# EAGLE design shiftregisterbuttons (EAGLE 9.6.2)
Assembly variants: CS HIGH, CS LOW
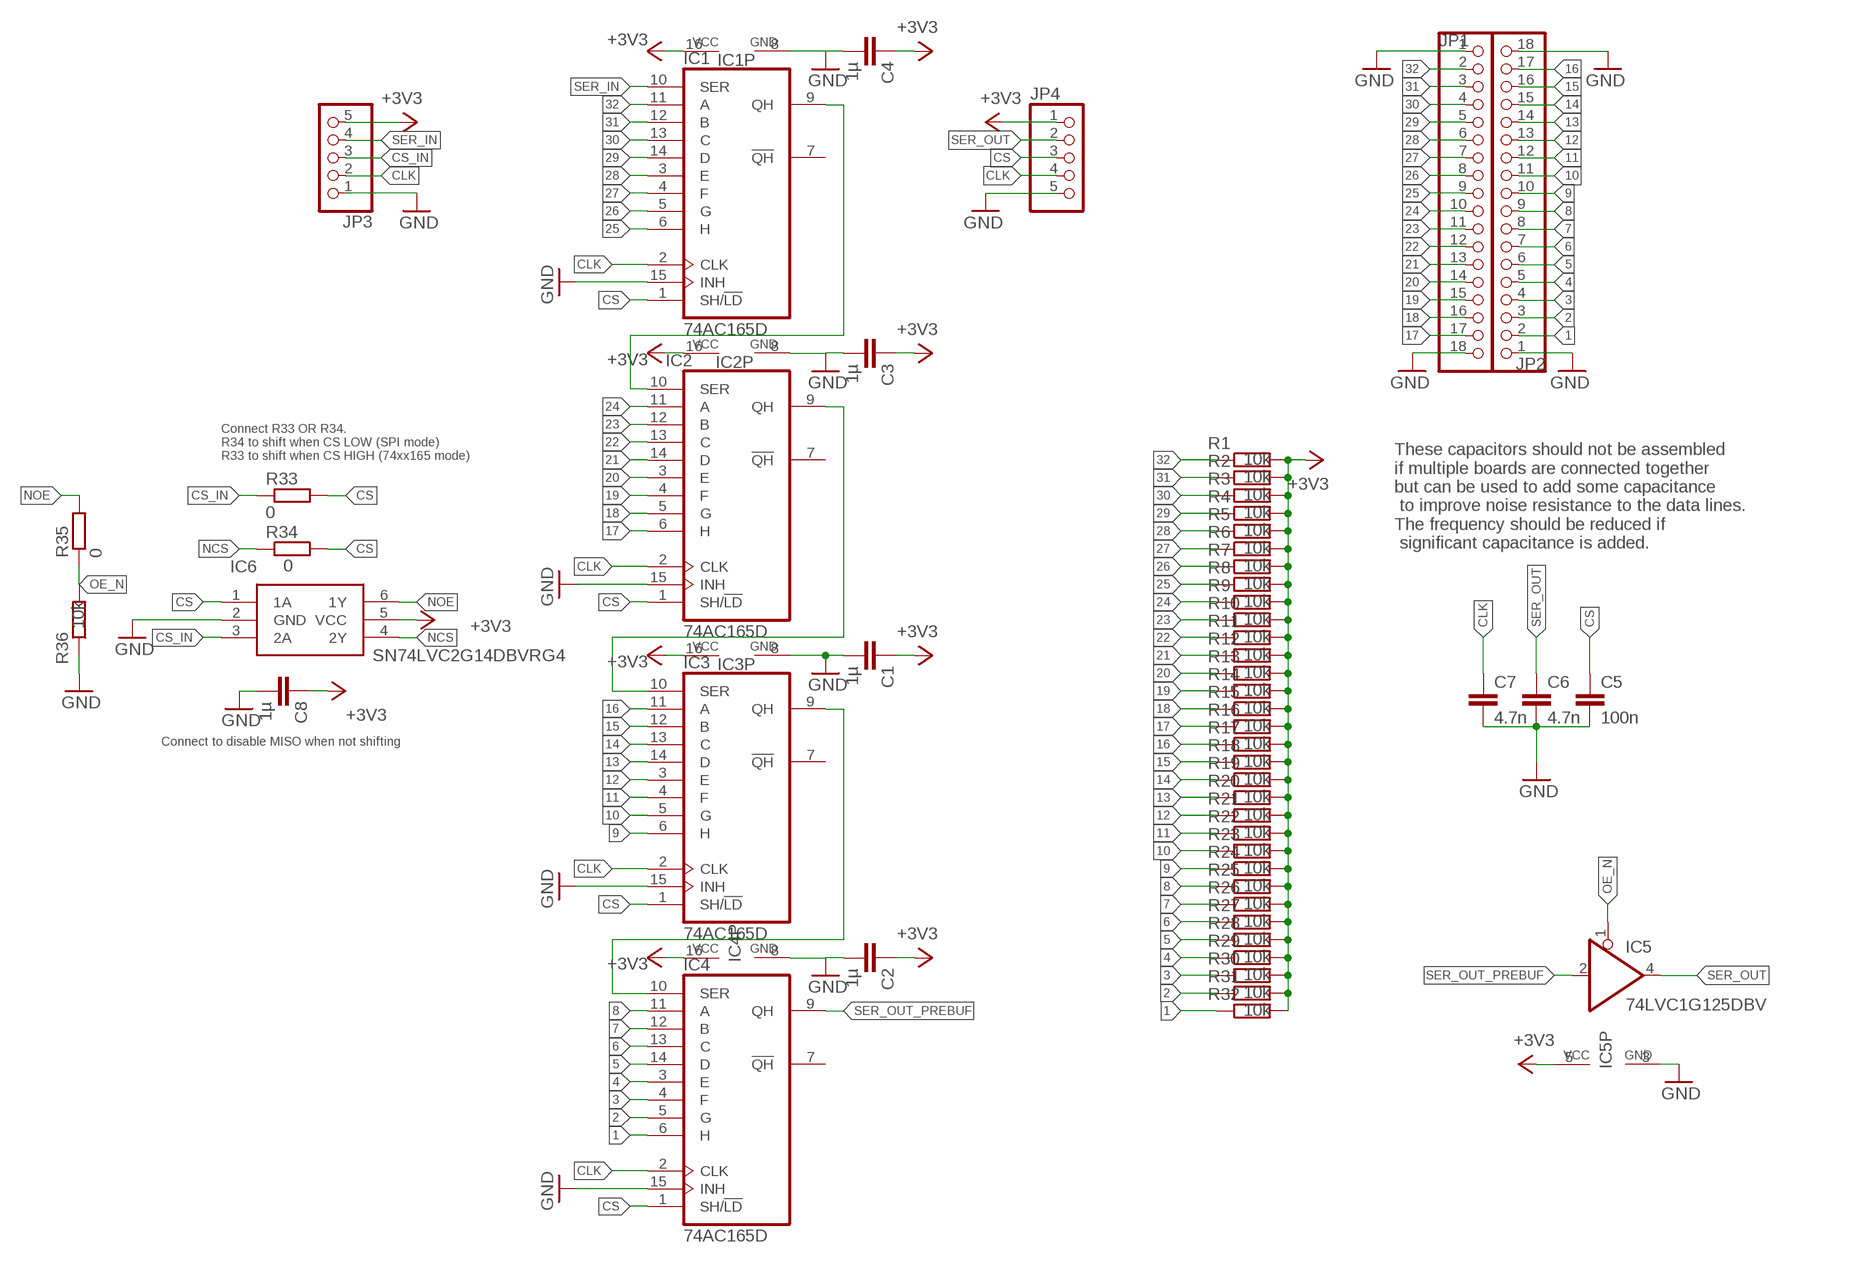
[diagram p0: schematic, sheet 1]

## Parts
C1  1µ  C-EUC0603  [C0603]
C2  1µ  C-EUC0603  [C0603]
C3  1µ  C-EUC0603  [C0603]
C4  1µ  C-EUC0603  [C0603]
C5  100n  C-EUC0603  [C0603]  (not fitted in variant CS HIGH)  (not fitted in variant CS LOW)
C6  4.7n  C-EUC0603  [C0603]  (not fitted in variant CS HIGH)  (not fitted in variant CS LOW)
C7  4.7n  C-EUC0603  [C0603]  (not fitted in variant CS HIGH)  (not fitted in variant CS LOW)
C8  1µ  C-EUC0603  [C0603]
IC1  74AC165D  [SO16]
IC2  74AC165D  [SO16]
IC3  74AC165D  [SO16]
IC4  74AC165D  [SO16]
IC5  74LVC1G125DBV  [SOT23-5]
IC6  SN74LVC2G14DBVRG4  [SOT95P280X145-6N]
JP1  PINHD-1X18  [1X18]
JP2  PINHD-1X18  [1X18]
JP3  PINHD-1X5  [1X05]
JP4  PINHD-1X5  [1X05]
R1  10k  R-EU_R0603  [R0603]
R2  10k  R-EU_R0603  [R0603]
R3  10k  R-EU_R0603  [R0603]
R4  10k  R-EU_R0603  [R0603]
R5  10k  R-EU_R0603  [R0603]
R6  10k  R-EU_R0603  [R0603]
R7  10k  R-EU_R0603  [R0603]
R8  10k  R-EU_R0603  [R0603]
R9  10k  R-EU_R0603  [R0603]
R10  10k  R-EU_R0603  [R0603]
R11  10k  R-EU_R0603  [R0603]
R12  10k  R-EU_R0603  [R0603]
R13  10k  R-EU_R0603  [R0603]
R14  10k  R-EU_R0603  [R0603]
R15  10k  R-EU_R0603  [R0603]
R16  10k  R-EU_R0603  [R0603]
R17  10k  R-EU_R0603  [R0603]
R18  10k  R-EU_R0603  [R0603]
R19  10k  R-EU_R0603  [R0603]
R20  10k  R-EU_R0603  [R0603]
R21  10k  R-EU_R0603  [R0603]
R22  10k  R-EU_R0603  [R0603]
R23  10k  R-EU_R0603  [R0603]
R24  10k  R-EU_R0603  [R0603]
R25  10k  R-EU_R0603  [R0603]
R26  10k  R-EU_R0603  [R0603]
R27  10k  R-EU_R0603  [R0603]
R28  10k  R-EU_R0603  [R0603]
R29  10k  R-EU_R0603  [R0603]
R30  10k  R-EU_R0603  [R0603]
R31  10k  R-EU_R0603  [R0603]
R32  10k  R-EU_R0603  [R0603]
R33  0  R-EU_R0603  [R0603]  (not fitted in variant CS LOW)
R34  0  R-EU_R0603  [R0603]  (not fitted in variant CS HIGH)
R35  0  R-EU_R0603  [R0603]
R36  10k  R-EU_R0603  [R0603]

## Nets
1: IC4.6(H) JP2.2 R32.1
2: IC4.5(G) JP2.3 R31.1
3: IC4.4(F) JP2.4 R30.1
4: IC4.3(E) JP2.5 R29.1
5: IC4.14(D) JP2.6 R28.1
6: IC4.13(C) JP2.7 R27.1
7: IC4.12(B) JP2.8 R26.1
8: IC4.11(A) JP2.9 R25.1
9: IC3.6(H) JP2.10 R24.1
10: IC3.5(G) JP2.11 R23.1
11: IC3.4(F) JP2.12 R22.1
12: IC3.3(E) JP2.13 R21.1
13: IC3.14(D) JP2.14 R20.1
14: IC3.13(C) JP2.15 R19.1
15: IC3.12(B) JP2.16 R18.1
16: IC3.11(A) JP2.17 R17.1
17: IC2.6(H) JP1.17 R16.1
18: IC2.5(G) JP1.16 R15.1
19: IC2.4(F) JP1.15 R14.1
20: IC2.3(E) JP1.14 R13.1
21: IC2.14(D) JP1.13 R12.1
22: IC2.13(C) JP1.12 R11.1
23: IC2.12(B) JP1.11 R10.1
24: IC2.11(A) JP1.10 R9.1
25: IC1.6(H) JP1.9 R8.1
26: IC1.5(G) JP1.8 R7.1
27: IC1.4(F) JP1.7 R6.1
28: IC1.3(E) JP1.6 R5.1
29: IC1.14(D) JP1.5 R4.1
30: IC1.13(C) JP1.4 R3.1
31: IC1.12(B) JP1.3 R2.1
32: IC1.11(A) JP1.2 R1.1
+3V3: C1.1 C2.1 C3.1 C4.1 C8.1 IC1.16(VCC) IC2.16(VCC) IC3.16(VCC) IC4.16(VCC) IC5.5(VCC) IC6.5(VCC) JP3.5 JP4.1 R1.2 R2.2 R3.2 R4.2 R5.2 R6.2 R7.2 R8.2 R9.2 R10.2 R11.2 R12.2 R13.2 R14.2 R15.2 R16.2 R17.2 R18.2 R19.2 R20.2 R21.2 R22.2 R23.2 R24.2 R25.2 R26.2 R27.2 R28.2 R29.2 R30.2 R31.2 R32.2
CLK: C7.1 IC1.2(CLK) IC2.2(CLK) IC3.2(CLK) IC4.2(CLK) JP3.2 JP4.4
CS: C5.1 IC1.1(SH/!LD) IC2.1(SH/!LD) IC3.1(SH/!LD) IC4.1(SH/!LD) IC6.1(1A) JP4.3 R33.2 R34.2
CS_IN: IC6.3(2A) JP3.3 R33.1
GND: C1.2 C2.2 C3.2 C4.2 C5.2 C6.2 C7.2 C8.2 IC1.8(GND) IC1.15(INH) IC2.8(GND) IC2.15(INH) IC3.8(GND) IC3.15(INH) IC4.8(GND) IC4.15(INH) IC5.3(GND) IC6.2(GND) JP1.1 JP1.18 JP2.1 JP2.18 JP3.1 JP4.5 R36.1
N$1: IC2.9(QH) IC3.10(SER)
N$2: IC3.9(QH) IC4.10(SER)
NCS: IC6.4(2Y) R34.1
NOE: IC6.6(1Y) R35.2
OE_N: IC5.1(OE) R35.1 R36.2
SER1: IC1.9(QH) IC2.10(SER)
SER_IN: IC1.10(SER) JP3.4
SER_OUT: C6.1 IC5.4(O) JP4.2
SER_OUT_PREBUF: IC4.9(QH) IC5.2(I)
Unconnected: IC1.7(!QH) IC2.7(!QH) IC3.7(!QH) IC4.7(!QH)

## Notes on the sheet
- Connect R33 OR R34.
  R34 to shift when CS LOW (SPI mode)
  R33 to shift when CS HIGH (74xx165 mode)
- These capacitors should not be assembled 
  if multiple boards are connected together 
  but can be used to add some capacitance
   to improve noise resistance to the data lines.
  The frequency should be reduced if
   significant capacitance is added.
- Connect to disable MISO when not shifting

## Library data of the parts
C1-C8 = resistor:C-EU: CAPACITOR, European symbol
IC1-IC4 = 74xx-eu:74*165: 8-bit parallel load SHIFT REGISTER
IC5 = 74xx-little-de:74*1G125: Single Bus Buffer Gate with 3-State Output
IC6 = SamacSys_Parts:SN74LVC2G14DBVRG4: Dual Schmitt-Trigger Inverter Source: Datasheet; ARROW_PART_NUMBER: SN74LVC2G14DBVRG4; ARROW_PRICE-STOCK: https://www.arrow.com/en/products/sn74lvc2g14dbvrg4/texas-instruments?utm_currency=USD&region=nac; DESCRIPTION: Dual Schmitt-Trigger Inverter; HEIGHT: 1.45mm; MANUFACTURER_NAME: Texas Instruments; MANUFACTURER_PART_NUMBER: SN74LVC2G14DBVRG4; MOUSER_PART_NUMBER: 595-SN74LVC2G14DBVG4; MOUSER_PRICE-STOCK: https://www.mouser.co.uk/ProductDetail/Texas-Instruments/SN74LVC2G14DBVRG4?qs=pajgIaoyDUjLahZkznp%2F9Q%3D%3D
JP1 JP2 = pinhead:PINHD-1X18: PIN HEADER
JP3 JP4 = pinhead:PINHD-1X5: PIN HEADER
R1-R36 = resistor:R-EU_: RESISTOR, European symbol

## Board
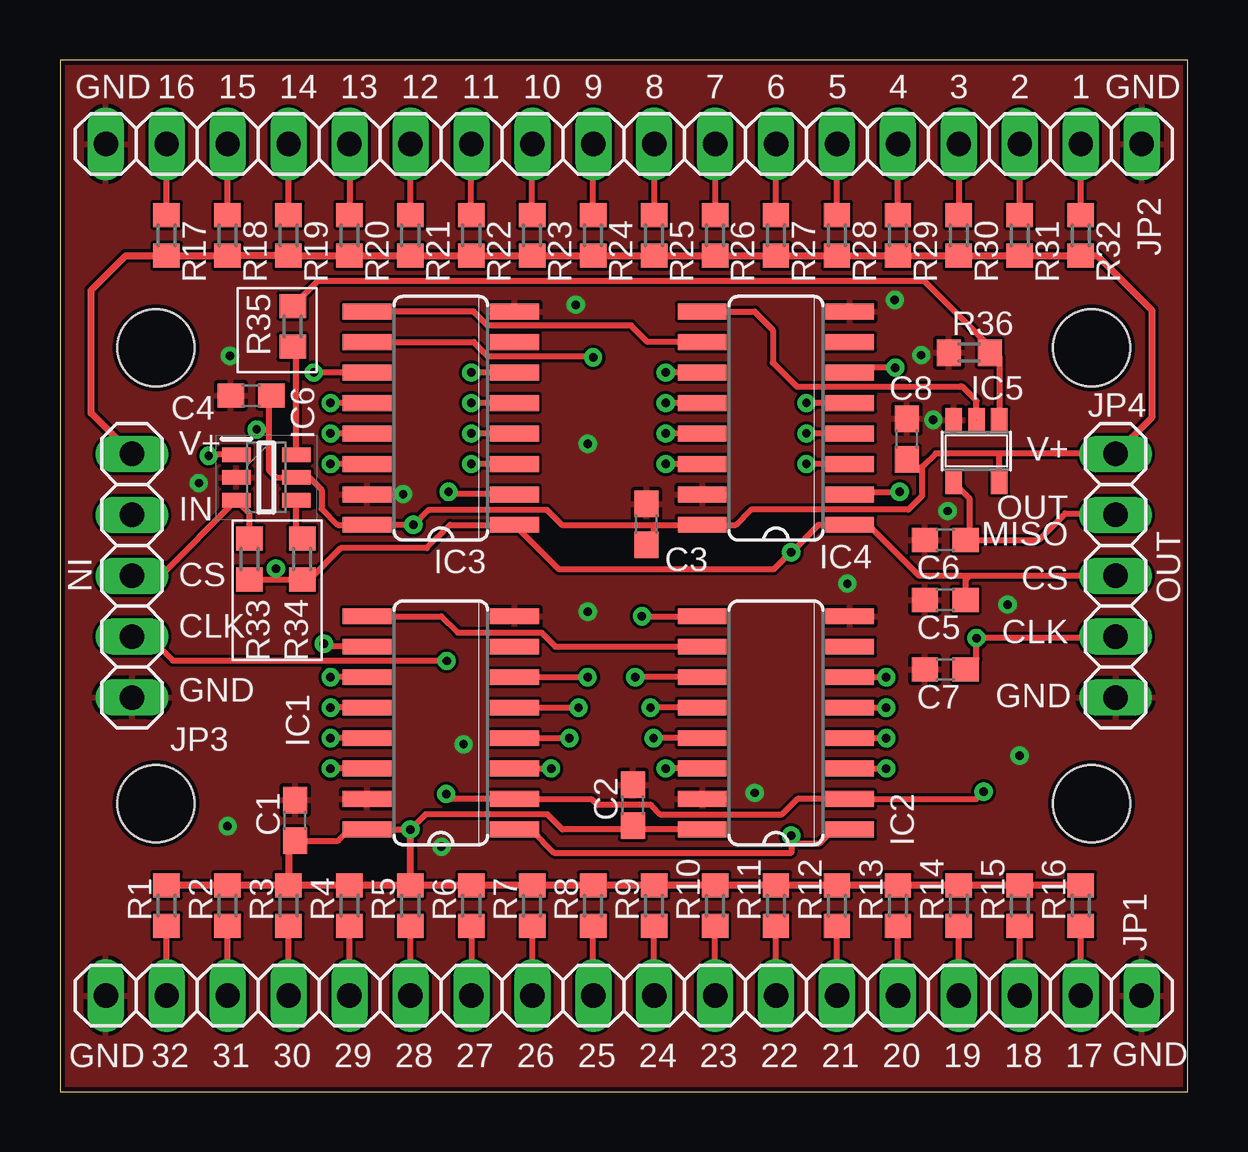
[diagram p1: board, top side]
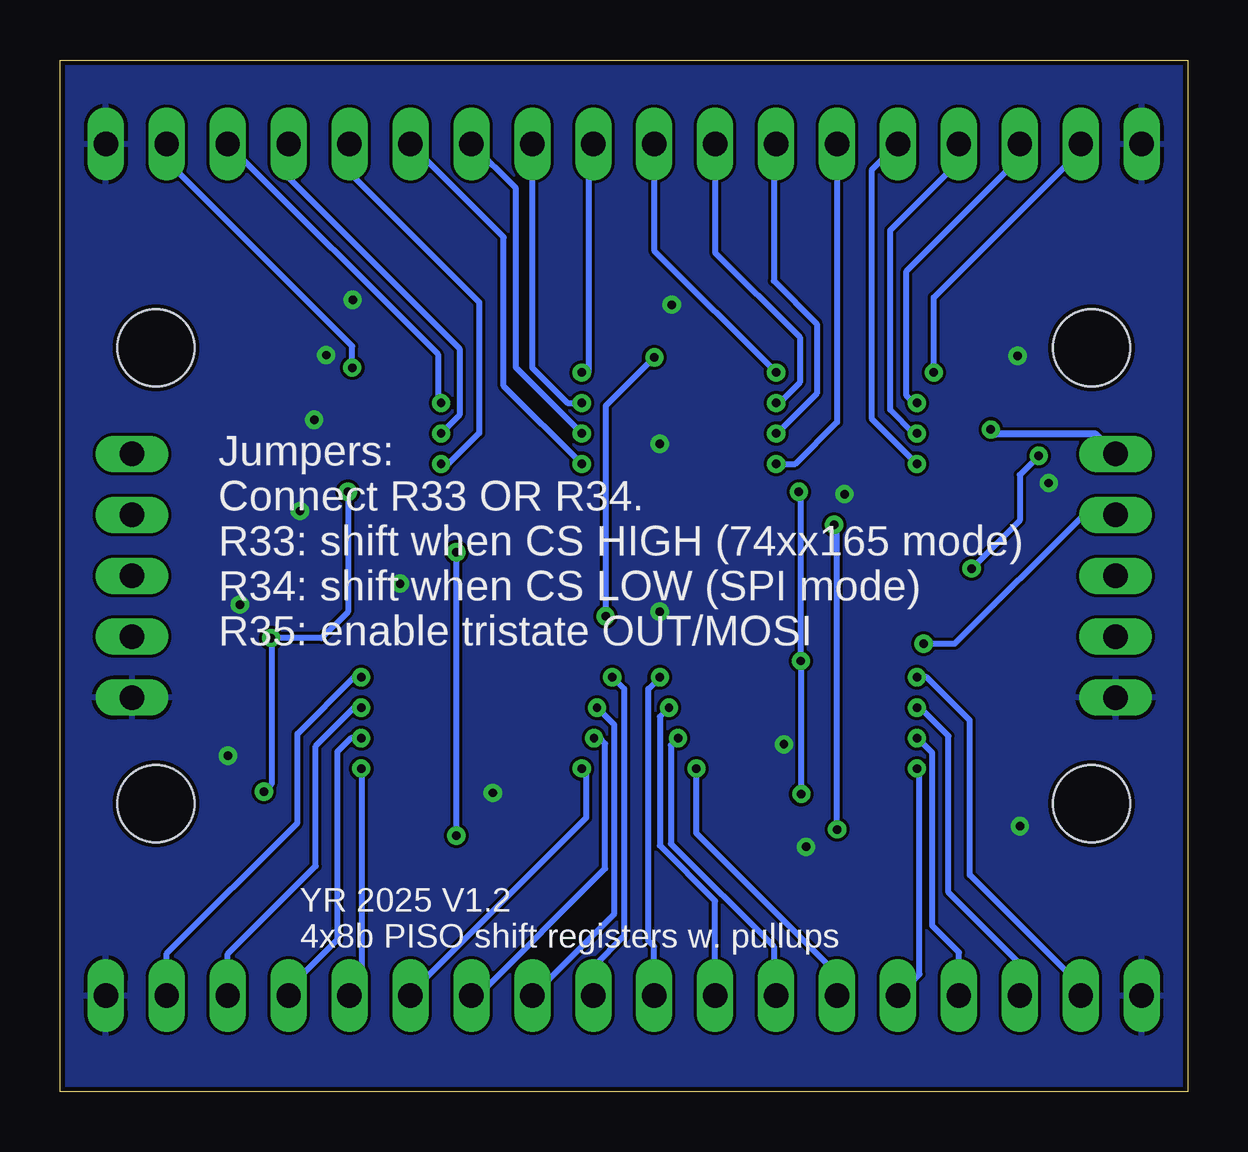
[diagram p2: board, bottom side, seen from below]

Size 47 x 43 mm. Coordinates in mm from the lower left corner, seen from the top.
Outline: 0,43 0,0 47,0 47,43 0,43
Copper layers (1*16): Top 0.035mm / dielectric 1.5mm / Bottom 0.035mm
Design rules "jlcpcb *": minimum track width 5mil, minimum drill 0.3mm, track to track 5mil, track to pad 5mil, pad to pad 5mil, via to via 5mil, smd to smd 5mil, copper to edge 0.2mm, drill to drill 8mil, minimum pad ring 10mil, minimum via ring 8mil, stop-mask expansion 4mil, vias tented up to drill 4mm, thermal gap 6mil
Holes 3.2 mm at 4,31 4,12 43,12 43,31

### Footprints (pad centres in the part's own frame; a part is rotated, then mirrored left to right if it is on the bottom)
C0603 = smd 1.1 x 1: 1 -0.85,0; 2 0.85,0
SO16 = smd 0.66 x 2.032: 1 -4.445,-3.073; 2 -3.175,-3.073; 3 -1.905,-3.073; 4 -0.635,-3.073; 5 0.635,-3.073; 6 1.905,-3.073; 7 3.175,-3.073; 8 4.445,-3.073; 9 4.445,3.073; 10 3.175,3.073; 11 1.905,3.073; 12 0.635,3.073; 13 -0.635,3.073; 14 -1.905,3.073; 15 -3.175,3.073; 16 -4.445,3.073
SOT23-5 = smd 0.69 x 0.99: 1 -0.95,-1.29; 2 0,-1.29; 3 0.95,-1.29; 4 0.95,1.3; 5 -0.95,1.3
SOT95P280X145-6N = smd 1.2 x 0.6: 1 -1.25,0.95; 2 -1.25,0; 3 -1.25,-0.95; 4 1.25,-0.95; 5 1.25,0; 6 1.25,0.95
1X18 = drill 1.016 long: 1 -21.59,0; 2 -19.05,0; 3 -16.51,0; 4 -13.97,0; 5 -11.43,0; 6 -8.89,0; 7 -6.35,0; 8 -3.81,0; 9 -1.27,0; 10 1.27,0; 11 3.81,0; 12 6.35,0; 13 8.89,0; 14 11.43,0; 15 13.97,0; 16 16.51,0; 17 19.05,0; 18 21.59,0
1X05 = drill 1.016 long: 1 -5.08,0; 2 -2.54,0; 3 0,0; 4 2.54,0; 5 5.08,0
R0603 = smd 1 x 1.1: 1 -0.85,0; 2 0.85,0

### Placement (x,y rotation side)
C1  9.79,11.3 90 top
C2  23.88,11.94 90 top
C3  24.44,23.65 90 top
C4  7.97,29.01 180 top
C5  36.9,20.5 180 top  (not fitted)
C6  36.9,23 180 top  (not fitted)
C7  36.9,17.6 180 top  (not fitted)
C8  35.3,27.2 90 top
IC1  15.88,15.37 90 top
IC2  29.84,15.37 90 top
IC3  15.88,28.07 90 top
IC4  29.84,28.07 90 top
IC5  38.2,26.7 180 top
IC6  8.6,25.6 0 top
JP1  23.5,4 0 top
JP2  23.5,39.5 180 top
JP3  3,21.5 90 top
JP4  44,21.5 270 top
R1  4.45,7.75 90 top
R2  6.99,7.75 90 top
R3  9.53,7.75 90 top
R4  12.06,7.75 90 top
R5  14.61,7.75 90 top
R6  17.14,7.75 90 top
R7  19.68,7.75 90 top
R8  22.23,7.75 90 top
R9  24.77,7.75 90 top
R10  27.3,7.75 90 top
R11  29.84,7.75 90 top
R12  32.38,7.75 90 top
R13  34.92,7.75 90 top
R14  37.47,7.75 90 top
R15  40.01,7.75 90 top
R16  42.55,7.75 90 top
R17  4.45,35.69 270 top
R18  6.99,35.69 270 top
R19  9.53,35.69 270 top
R20  12.06,35.69 270 top
R21  14.61,35.69 270 top
R22  17.14,35.69 270 top
R23  19.68,35.69 270 top
R24  22.23,35.69 270 top
R25  24.77,35.69 270 top
R26  27.3,35.69 270 top
R27  29.84,35.69 270 top
R28  32.38,35.69 270 top
R29  34.92,35.69 270 top
R30  37.47,35.69 270 top
R31  40.01,35.69 270 top
R32  42.55,35.69 270 top
R33  7.9,22.2 270 top
R34  10.1,22.2 270 top  (not fitted)
R35  9.7,31.9 270 top
R36  37.9,30.8 0 top

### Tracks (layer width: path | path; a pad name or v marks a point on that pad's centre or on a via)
1  (via drill 0.35)
  Top 0.254: IC4.6 33.12,30.17 v34.82,30.17 | R32.1 42.37,36.72 42.55,36.9 JP2.2
  Bottom 0.254: v34.82,30.17 34.82,31.07 42.55,38.8 JP2.2
2  (via drill 0.35)
  Top 0.254: IC4.5 v31.11,28.7 | R31.1 40.09,36.62 40.01,36.7 JP2.3
  Bottom 0.254: JP2.3 31.24,30.73 31.24,28.83 v31.11,28.7
3  (via drill 0.35)
  Top 0.254: IC4.4 v31.11,27.43 | JP2.4 R30.1
  Bottom 0.254: JP2.4 37.47,38.1 30.34,30.98 30.34,28.2 v31.11,27.43
4  (via drill 0.35)
  Top 0.254: IC4.3 v31.11,26.16 | R29.1 34.9,36.57 34.93,36.6 JP2.5
  Bottom 0.254: JP2.5 34.93,38.3 29.53,32.9 29.53,27.45 30.82,26.16 v31.11,26.16
5  (via drill 0.35)
  Top 0.254: IC4.14 v25.25,26.16 | R28.1 32.38,36.41 32.39,36.4 JP2.6
  Bottom 0.254: v25.25,26.16 28.5,29.42 28.5,35.61 JP2.6
6  (via drill 0.35)
  Top 0.254: IC4.13 v25.25,27.43 | R27.1 29.84,39.34 29.93,39.42 JP2.7
  Bottom 0.254: v25.25,27.43 27.99,30.18 27.99,37.65 JP2.7 | JP2.7
7  (via drill 0.35)
  Top 0.254: IC4.12 v25.25,28.7 | JP2.8 27.31,36.9 27.13,36.72 R26.1
  Bottom 0.254: JP2.8 27.31,30.16 25.85,28.7 v25.25,28.7
8  (via drill 0.35)
  Top 0.254: IC4.11 v25.25,29.97 | JP2.9 24.77,36.8 24.64,36.67 R25.1
  Bottom 0.254: JP2.9 24.97,39.3 24.97,29.97 v25.25,29.97
9  (via drill 0.35)
  Top 0.254: IC3.6 v17.14,29.97 | R24.1 JP2.10
  Bottom 0.254: JP2.10 22.23,35.06 v17.14,29.97
10  (via drill 0.35)
  Top 0.254: JP2.11 19.64,39.45 19.68,39.4 R23.1 | IC3.5 v17.14,28.7
  Bottom 0.254: JP2.11 19.69,34.97 16.16,31.44 16.16,29.56 17.01,28.7 v17.14,28.7
11  (via drill 0.35)
  Top 0.254: IC3.4 v17.14,27.43 | R22.1 JP2.12
  Bottom 0.254: JP2.12 17.25,39.4 17.25,33.8 15.45,32 15.45,29.1 17.12,27.43 v17.14,27.43
12  (via drill 0.35)
  Top 0.254: IC3.3 v17.14,26.16 | R21.1 JP2.13
  Bottom 0.254: v17.14,26.16 16.34,26.16 14.61,27.9 JP2.13
13  (via drill 0.35)
  Top 0.254: IC3.14 v11.28,26.16 | JP2.14 R20.1
  Bottom 0.254: v11.28,26.16 13.17,28.06 13.17,38.4 JP2.14
14  (via drill 0.35)
  Top 0.254: IC3.13 v11.28,27.43 | R19.1 JP2.15
  Bottom 0.254: v11.28,27.43 11.4,27.43 12.39,28.42 12.39,35.9 9.53,38.76 JP2.15
15  (via drill 0.35)
  Top 0.254: JP2.16 | IC3.12 v11.28,28.7 | R18.1 JP2.16
  Bottom 0.254: v11.28,28.7 11.4,28.7 11.71,29.01 11.71,34.2 7.09,38.82 7.09,39.5 JP2.16
16  (via drill 0.35)
  Top 0.254: JP2.17 R17.1 | IC3.11 v10.58,29.97
  Bottom 0.254: v10.58,29.97 10.58,33.1 4.45,39.23 JP2.17
17  (via drill 0.35)
  Top 0.254: IC2.6 v34.44,17.27 | JP1.17 R16.1
  Bottom 0.254: JP1.17 42.55,5.75 37.1,11.2 37.1,14.91 34.74,17.27 v34.44,17.27
18  (via drill 0.35)
  Top 0.254: IC2.5 v34.44,16 | JP1.16 R15.1
  Bottom 0.254: JP1.16 40.01,5.73 36.34,9.4 36.34,14.4 34.74,16 v34.44,16
19  (via drill 0.35)
  Top 0.254: IC2.4 v34.44,14.73 | JP1.15 R14.1
  Bottom 0.254: v34.44,14.73 34.87,14.73 35.43,14.17 35.43,6.34 37.47,4.3 JP1.15
20  (via drill 0.35)
  Top 0.254: IC2.3 v34.44,13.46 | JP1.14 R13.1
  Bottom 0.254: JP1.14 34.42,4 34.42,13.44 v34.44,13.46
21  (via drill 0.35)
  Top 0.254: IC2.14 v25.25,13.46 | JP1.13 R12.1
  Bottom 0.254: v25.25,13.46 25.07,13.28 25.07,11.41 32.39,4.09 JP1.13
22  (via drill 0.35)
  Top 0.254: IC2.13 v24.74,14.73 | JP1.12 R11.1
  Bottom 0.254: JP1.12 29.58,4 24.28,9.3 24.28,14.5 24.51,14.73 v24.74,14.73
23  (via drill 0.35)
  Top 0.254: IC2.12 v24.61,16 | JP1.11 R10.1
  Bottom 0.254: v24.61,16 23.89,15.28 23.89,7.42 JP1.11
24  (via drill 0.35)
  Top 0.254: IC2.11 v23.98,17.27 | JP1.10 R9.1
  Bottom 0.254: JP1.10 24.77,5.2 23.49,6.48 23.49,16.78 v23.98,17.27
25  (via drill 0.35)
  Top 0.254: IC1.6 v22,17.27 | JP1.9 R8.1
  Bottom 0.254: v22,17.27 22.48,16.79 22.48,6.29 22.23,6.04 JP1.9
26  (via drill 0.35)
  Top 0.254: IC1.5 v21.61,16 | JP1.8 R7.1
  Bottom 0.254: JP1.8 19.69,7.95 21.99,10.25 21.99,15.62 v21.61,16
27  (via drill 0.35)
  Top 0.254: IC1.4 v21.23,14.73 | JP1.7 R6.1
  Bottom 0.254: JP1.7 17.25,4.1 17.25,6.05 21.53,10.33 21.53,14.44 v21.23,14.73
28  (via drill 0.35)
  Top 0.254: IC1.3 v20.47,13.46 | JP1.6 R5.1
  Bottom 0.254: JP1.6 14.61,4.9 20.47,10.76 v20.47,13.46
29  (via drill 0.35)
  Top 0.254: IC1.14 v11.28,13.46 | JP1.5 R4.1
  Bottom 0.254: v11.28,13.46 11.18,13.36 11.18,4.89 JP1.5
30  (via drill 0.35)
  Top 0.254: IC1.13 v11.28,14.73 | JP1.4 R3.1
  Bottom 0.254: v11.28,14.73 11.25,14.73 10.64,14.12 10.64,6.92 9.53,5.8 JP1.4
31  (via drill 0.35)
  Top 0.254: IC1.12 v11.28,16 | JP1.3 R2.1
  Bottom 0.254: v11.28,16 11.15,16 9.96,14.81 9.96,8.3 6.99,5.33 JP1.3
32  (via drill 0.35)
  Top 0.254: IC1.11 v11.28,17.27 | JP1.2 R1.1
  Bottom 0.254: v11.28,17.27 10.88,17.27 9.08,15.47 9.08,9.03 4.45,4.4 JP1.2
+3V3  (via drill 0.35)
  Top 0.254: IC2.16 23.71,10.92 | 23.71,10.92 20.95,10.92 20.32,11.56 15.24,11.56 v14.61,10.92 IC1.16 12.76,10.96 12.1,10.96 11.6,10.45 C1.1 | 24.77,23.62 20.92,23.62 20.29,24.26 15.37,24.26 v14.73,23.62 IC3.16 11.58,23.62 10.9,24.3 10.9,25.1 10.4,25.6 IC6.5 9,25.6 8.7,25.9 8.7,27.6 | 24.77,23.62 IC4.16 28.17,23.62 28.8,24.26 35.36,24.26 35.93,24.83 35.93,26.03 | C3.1 24.77,23.13 24.77,23.62 | C2.1 23.71,10.92 | JP4.1 43.98,26.6 39.2,26.6 | 39.2,26.6 36.5,26.6 35.93,26.03 | IC5.5 39.15,26.55 39.2,26.6 | 8.7,27.6 8.7,28.89 C4.1 8.6,29.23 | v8.2,27.6 8.7,27.6 | C8.1 35.62,26.03 35.93,26.03
  Top 0.3: JP4.1 45.5,28.08 45.5,32.58 43.24,34.84 R32.2 R31.2 R30.2 R29.2 R28.2 R27.2 R26.2 R25.2 R24.2 R23.2 R22.2 R21.2 R20.2 R19.2 R18.2 R17.2 2.74,34.84 1.3,33.4 1.3,28.28 JP3.5 | R16.2 R15.2 R14.2 R13.2 R12.2 R11.2 R10.2 R9.2 R8.2 R7.2 R6.2 R5.2 | R5.2 v14.61,10.92 | R5.2 R4.2 R3.2 | C1.1 9.53,10.18 R3.2 | R3.2 R2.2 R1.2
  Bottom 0.254: v14.61,10.92 14.61,23.5 v14.73,23.62
  Bottom 0.3: JP3.5 3.82,27.4 8,27.4 v8.2,27.6
CLK  (via drill 0.35)
  Top 0.254: 43,18.96 JP4.4 43.94,18.9 v38.2,18.9 38.2,18.05 C7.1 | JP3.2 3.71,18.96 4.71,17.96 16.11,17.96 v16.12,17.95 | v16.2,25 16.3,24.9 IC3.2 | IC4.2 33.03,25 v35,25 | v16.1,12.4 16.31,12.19 IC1.2 22.15,12.19 22.4,11.94 24.64,11.94 25.02,11.56 30.1,11.56 30.73,12.19 IC2.2 38.19,12.19 v38.5,12.5
  Bottom 0.254: v16.2,25 16.12,24.92 v16.12,17.95 16.1,17.93 v16.1,12.4 | v35,25 35,20 36.1,18.9 v38.2,18.9 38.18,18.88 38.18,12.82 v38.5,12.5
CS  (via drill 0.35)
  Top 0.254: JP4.3 37.9,21.5 | 37.9,21.5 35.83,21.5 33.7,23.62 IC4.1 31.62,23.62 v30.48,22.48 30.46,22.48 29.75,21.77 20.8,21.77 IC3.1 16.26,23.62 15.29,22.65 11.7,22.65 10.4,21.35 R34.2 9,21.35 | IC1.1 19.63,10.92 20.6,9.96 30.48,9.96 30.48,10.34 | 30.48,10.34 31.65,10.34 32.23,10.92 IC2.1 | v30.48,10.67 30.48,10.34 | C5.1 37.75,21.35 37.9,21.5 | R33.2 9,21.35 | IC6.1 6.25,26.55 v6.2,26.5 | v9,21.8 9,21.35
  Bottom 0.254: v30.48,22.48 v30.48,10.67 | v6.2,26.5 7,25.7 7,23.8 v9,21.8
CS_IN
  Top 0.254: JP3.3 4.2,21.5 IC6.3 7.9,24.1 R33.1
GND  (via drill 0.35)
  Top 0.254: C2.2 23.91,12.82 | IC3.15 v14.29,24.89 v14.3,24.9
  other vias: 22,27 22,20 39.5,20.3 37,24.2 36.4,28 40,14 28.96,12.45 16.82,14.47 6.99,11.06 5.79,25.36 7.08,30.66 15.9,10.2 21.5,32.8 34.8,33 35.9,30.7 32.82,21.17
  pour Bottom: 0,43.18 0,-0.27 47,-0.27 47,43.18
  pour Top: 0,43.18 0,-0.27 47,-0.27 47,43.18
N$1  (via drill 0.35)
  Top 0.254: IC3.10 17.24,31.24 17.83,30.66 22.17,30.66 v22.23,30.61 | v24.26,19.81 IC2.9
  Bottom 0.254: v22.23,30.61 24.26,28.57 v24.26,19.81
N$2
  Top 0.254: IC4.10 24.49,31.24 23.8,31.93 17.83,31.93 17.24,32.51 IC3.9
NCS
  Top 0.254: R34.1 9.85,23.3 IC6.4
NOE
  Top 0.254: IC6.6 9.85,30.9 R35.2
OE_N
  Top 0.254: R35.1 10.75,33.8 36,33.8 38.9,30.9 | 38.9,30.9 39.15,30.65 IC5.1 | R36.2 38.85,30.9 38.9,30.9
SER1
  Top 0.254: IC1.9 15.9,19.81 16.59,19.13 20.07,19.13 20.65,18.54 IC2.10
SER_IN  (via drill 0.35)
  Top 0.254: IC1.10 11.13,18.54 v11,18.67
  Bottom 0.254: v11,18.67 9.7,18.67 4.33,24.04 JP3.4
SER_OUT
  Top 0.254: IC5.4 37.9,24.75 37.9,23.15 C6.1 40.8,23 41.9,24.1 43.94,24.1 JP4.2
SER_OUT_PREBUF
  Top 0.254: IC4.9 28.96,32.51 29.72,31.75 29.72,30.38 30.72,29.38 37.5,29.38 37.62,29.38 38.2,28.8 IC5.2

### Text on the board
tPlace: GND | 16 | 15 | 14 | 13 | 12 | 11 | 10 | 9 | 8 | 7 | 6 | 5 | 4 | 3 | 2 | 1 | GND | V+ | V+ | OUT | IN | MISO | OUT | IN | CS | CS | CLK | CLK | GND | GND | GND | 32 | 31 | 30 | 29 | 28 | 27 | 26 | 25 | 24 | 23 | 22 | 21 | 20 | 19 | 18 | 17 | GND
bPlace: Jumpers: / Connect R33 OR R34. / R33: shift when CS HIGH (74xx165 mode) / R34: shift when CS LOW (SPI mode) / R35: enable tristate OUT/MOSI | YR 2025 V1.2 / 4x8b PISO shift registers w. pullups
